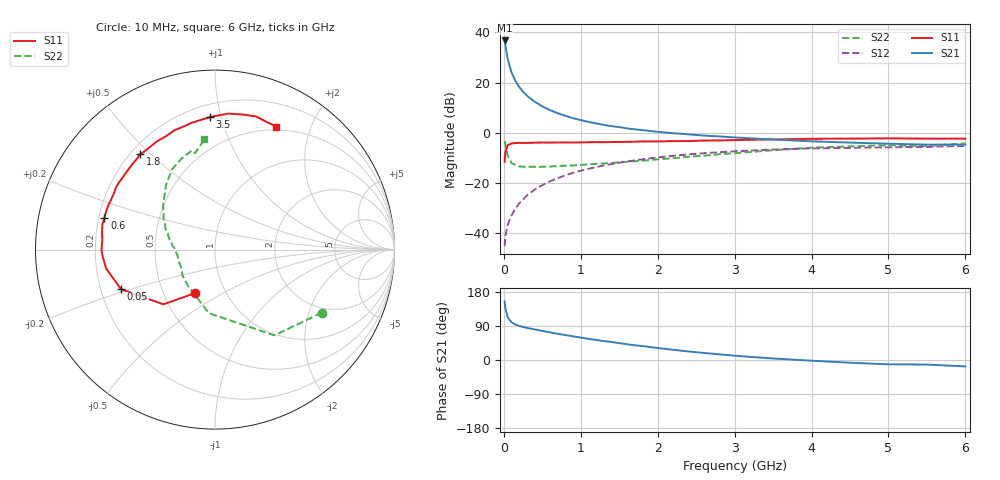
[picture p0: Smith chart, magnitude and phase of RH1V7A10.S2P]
! SIEMENS Small Signal Semiconductors
! BFR106
! Si NPN RF Bipolar Junction Transistor in SOT23
! VCE = 1.75 V  IC = 100 mA
! Common Emitter S-Parameters:  August  1996
# GHz  S  MA  R  50
!  f  S11  S21  S12  S22
! GHz  MAG  ANG  MAG  ANG  MAG  ANG  MAG  ANG
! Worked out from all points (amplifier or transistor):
!   36 points, 10 MHz to 6 GHz, reference 50 ohm
!   highest |S21| = 36.7 dB at 10 MHz (marker M1)
!   |S21| within 3 dB of that: start of sweep to 26.1 MHz
!   unconditionally stable (mu >= 1): 97.06 MHz to end of sweep
!   at 250 MHz: K = 1.18, MAG = 18.8 dB, |S12| = -26.4 dB
!   at 1.4 GHz: K = 1.14, MAG = 5.3 dB, |S12| = -12.4 dB
!   at 6 GHz: K = 1.03, MAG = -0.8 dB, |S12| = -5.2 dB
!   S11 on the Smith chart (normalised r, x): 10 MHz: 0.72, -0.38; 50 MHz: 0.29, -0.19; 600 MHz: 0.22, +0.13; 1.8 GHz: 0.24, +0.46; 3.5 GHz: 0.28, +0.92; 6 GHz: 0.46, +1.52
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0.01  0.2653 -114.3  68.5 154.4  0.0056 69.9  0.6912 -30.6
0.02  0.4189 -133.3  55 136.5  0.009 61.1  0.5814 -55.3
0.05  0.5682 -157.2  29.61 112.4  0.0148 57.9  0.3557 -95.5
0.1  0.6155 -170.1  15.86 99.6  0.0229 63.4  0.2519 -126.8
0.15  0.6269 -176.4  10.76 93.8  0.0312 68.1  0.2307 -142.0
0.2  0.6324 -179.8  8.16 90.0  0.0396 70.7  0.2152 -150.3
0.25  0.6307 177.5  6.521 87.1  0.0479 72.0  0.212 -157.4
0.3  0.63 175.2  5.475 84.9  0.0568 73.0  0.2122 -160.9
0.4  0.637 171.1  4.165 80.8  0.0746 73.0  0.2113 -167.0
0.5  0.6429 167.5  3.359 76.8  0.0913 72.6  0.2116 -171.3
0.6  0.6409 163.9  2.829 72.9  0.1087 71.3  0.214 -173.8
0.7  0.6426 160.6  2.461 69.0  0.126 70.2  0.2189 -176.3
0.8  0.6437 157.7  2.177 65.8  0.1436 68.6  0.2232 -179.0
0.9  0.6424 154.3  1.956 62.5  0.1605 66.9  0.2249 178.4
1.1  0.6509 148.0  1.652 55.9  0.1928 63.7  0.2369 175.1
1.4  0.6556 139.3  1.356 47.6  0.2401 58.3  0.2526 169.2
1.8  0.6758 128.2  1.135 36.8  0.2974 51.0  0.2782 161.1
2.2  0.6843 118.4  0.983 27.0  0.35 43.8  0.3129 152.9
3.5  0.7391 92.1  0.735 4.0  0.4666 21.8  0.4511 127.2
4.5  0.7681 78.4  0.64 -7.2  0.5037 7.7  0.54 110.3
5.5  0.7666 67.5  0.583 -12.1  0.5254 -0.6  0.5481 101.8
6  0.7661 63.5  0.586 -16.9  0.5502 -7.1  0.6172 95.5
